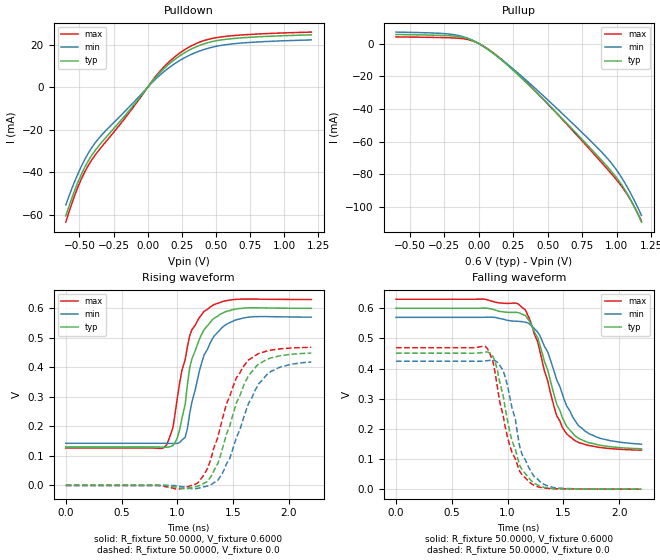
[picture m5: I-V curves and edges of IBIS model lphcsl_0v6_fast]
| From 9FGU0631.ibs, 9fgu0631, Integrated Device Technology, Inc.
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[Model]  lphcsl_0v6_fast
Model_type Output
Polarity   Non-Inverting
Enable   Active-High
Vmeas =  0.4000V
Cref =   2.0000pF
Rref =   0.0
Vref =   0.4000V
C_comp   1.1000pF   1.0000pF   1.2000pF
[Temperature Range]   25.0000   75.0000   0.0
[Voltage Range]   0.6000V   0.5700V   0.6300V
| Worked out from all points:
|   slope of the pulldown table from 0 to 0.09 V, typ, clamps not added: 13.2 ohm
|   slope of the pullup table from 0 to 0.09 V, typ, clamps not added: 17.6 ohm
|   rising waveform, R_fixture 50.0000, V_fixture 0.6000: 20-80 % time 171ps typ, 193ps min, 160ps max; typ from 0.13 V to 0.6 V
|   rising waveform, R_fixture 50.0000, V_fixture 0.0: 20-80 % time 243ps typ, 258ps min, 245ps max; typ from 0 V to 0.448 V
|   falling waveform, R_fixture 50.0000, V_fixture 0.6000: 20-80 % time 241ps typ, 278ps min, 235ps max; typ from 0.6 V to 0.134 V
|   falling waveform, R_fixture 50.0000, V_fixture 0.0: 20-80 % time 174ps typ, 171ps min, 183ps max; typ from 0.451 V to 0 V
[Pulldown]
|Voltage   I(typ)   I(min)   I(max)
-600mV    -60.47mA   -55.34mA   -63.45mA
-540mV    -49.36mA   -45.1mA    -51.8mA
-500mV    -42.97mA   -39.12mA   -45.21mA
-440mV    -35.14mA   -31.55mA   -37.31mA
-380mV    -29.3mA    -25.74mA   -31.48mA
-140mV    -11.3mA    -9.552mA   -12.37mA
60mV      4.726mA    3.957mA    5.199mA
220mV     14.11mA    12mA       15.38mA
360mV     19.15mA    16.55mA    20.68mA
500mV     21.85mA    19.24mA    23.3mA
740mV     23.48mA    21.06mA    24.82mA
1.2V      24.65mA    22.28mA    25.96mA
[Pullup]
|Voltage   I(typ)   I(min)   I(max)
-600mV    5.539mA    7.002mA    4.049mA
-160mV    4.38mA     5.132mA    3.309mA
-40mV     1.727mA    1.805mA    1.473mA
100mV     -5.748mA   -5.607mA   -5.36mA
240mV     -15.68mA   -14.9mA    -15.23mA
420mV     -30.15mA   -28.26mA   -30.01mA
740mV     -57.84mA   -53.76mA   -58.73mA
920mV     -74.2mA    -69.1mA    -75.68mA
1V        -82.24mA   -77.52mA   -83.58mA
1.06V     -89.61mA   -85.43mA   -90.31mA
1.12V     -98.68mA   -94.71mA   -98.6mA
1.18V     -109.4mA   -105.3mA   -108.8mA
[Ramp]
| variable   typ   min   max
dV/dt_r  0.2691/0.2450n   0.2510/0.2570n   0.2808/0.2412n
dV/dt_f  0.2797/0.2404n   0.2524/0.2723n   0.3004/0.2282n
R_load = 50.0000
[Rising Waveform]
R_fixture= 50.0000
V_fixture= 0.6000
V_fixture_min= 0.5700
V_fixture_max= 0.6300
|time   V(typ)   V(min)   V(max)
0s        130.4mV    142.8mV    126.9mV
870ps     130.1mV    142.8mV    126.5mV
960ps     134.6mV    142.1mV    195.7mV
1.04ns    226.2mV    153.4mV    388.9mV
1.07ns    274.7mV    163.4mV    426.6mV
1.11ns    398.7mV    242.9mV    506.9mV
1.24ns    528.2mV    442.6mV    590.2mV
1.33ns    567.1mV    506.5mV    612.8mV
1.53ns    598.2mV    561.7mV    630.6mV
2.2ns     600.2mV    570.4mV    630.1mV
[Rising Waveform]
R_fixture= 50.0000
V_fixture= 0.0
V_fixture_min= 0.0
V_fixture_max= 0.0
|time   V(typ)   V(min)   V(max)
0s        0V         0V         0V
1.02ns    -8.389mV   -3.022mV   -11.98mV
1.18ns    -2.49mV    -9.945mV   7.99mV
1.27ns    13.33mV    -1.936mV   57.87mV
1.4ns     119.8mV    38.53mV    220.3mV
1.53ns    281.2mV    163.6mV    365.4mV
1.62ns    359.3mV    259.4mV    417.3mV
1.73ns    411.4mV    345.2mV    446.9mV
1.84ns    432.3mV    386.8mV    458.7mV
2.2ns     448.5mV    418.4mV    468mV
[Falling Waveform]
R_fixture= 50.0000
V_fixture= 0.6000
V_fixture_min= 0.5700
V_fixture_max= 0.6300
|time   V(typ)   V(min)   V(max)
0s        600mV      570mV      630mV
1.09ns    586.1mV    556.8mV    615.3mV
1.16ns    576.3mV    553.7mV    594.4mV
1.29ns    477.3mV    508.5mV    456.9mV
1.36ns    394.8mV    455.2mV    359.1mV
1.44ns    282.5mV    362.9mV    244.4mV
1.53ns    208.1mV    275.8mV    183.2mV
1.64ns    167.7mV    209.1mV    154.3mV
1.73ns    154mV      183.8mV    144.7mV
2.2ns     133.9mV    149.3mV    129.4mV
[Falling Waveform]
R_fixture= 50.0000
V_fixture= 0.0
V_fixture_min= 0.0
V_fixture_max= 0.0
|time   V(typ)   V(min)   V(max)
0s        451.1mV    424.4mV    469.3mV
820ps     455.1mV    426.3mV    466.4mV
890ps     421mV      425.6mV    382.4mV
960ps     310.6mV    393.5mV    244.3mV
1.02ns    189.5mV    305.8mV    144.8mV
1.07ns    131.8mV    232.3mV    100.4mV
1.11ns    77.62mV    139.5mV    58.37mV
1.22ns    25.36mV    52.58mV    16.51mV
1.42ns    2.384mV    5.184mV    1.704mV
2.2ns     127.3uV    222.8uV    91.03uV
